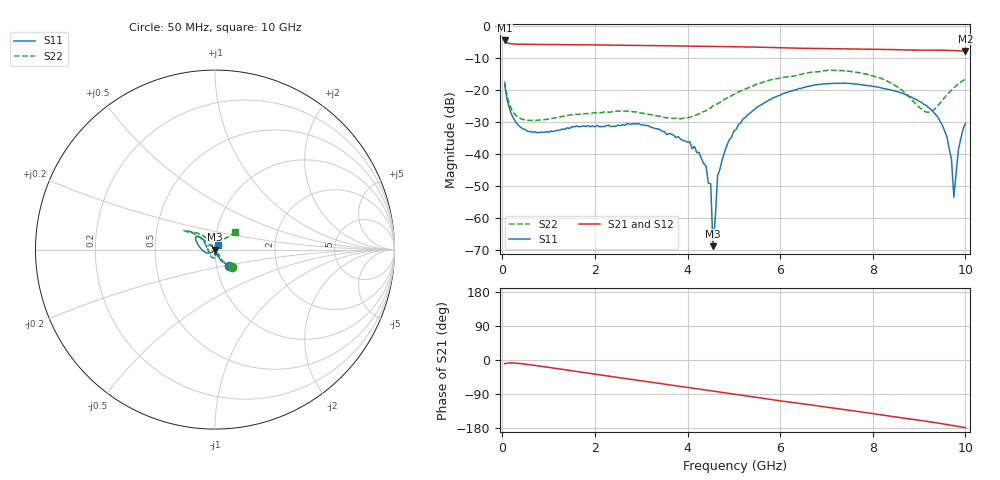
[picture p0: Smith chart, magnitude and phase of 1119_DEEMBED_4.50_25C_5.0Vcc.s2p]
!Hittite Microwave Corp.
!Digital Attenuator/PhaseShifter Rev 1.4.0
!Filename: C:\DATA\DATA\1119_DEEMBED_4.50_25C_5.0Vcc.s2p
!VNA ID: Agilent Technologies,N5224A,MY51441122,A.10.45.03
!Device type:
!2 Port Calibration.
!Temp(C): 25
!Lot Number:
!Serial Number:
!Operator:
!Misc:
!Attenuator:  4.500
# GHZ S DB R 50.0
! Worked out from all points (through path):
!   200 points, 50 MHz to 10 GHz, reference 50 ohm
!   highest |S21| = -4.50 dB at 50 MHz (marker M1); lowest = -7.8 dB at 10 GHz (marker M2)
!   group delay of S21, straight-line fit = 48.3 ps
!   lowest |S11| = -68.9 dB at 4.55 GHz (marker M3), VSWR 1.00, Z = 50 - j0.033 ohm
!   |S11| at or under -10 dB: start of sweep to end of sweep
!   |S22| runs from -29.5 to -13.8 dB; largest |S21 - S12| = 0.0013
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0.05  -18.28 -48.8  -4.50 -9.7  -4.50 -9.7  -17.41 -45.3
0.2  -27.69 -63.4  -5.56 -7.7  -5.56 -7.7  -26.08 -55.2
0.55  -33.00 -58.9  -5.71 -11.8  -5.71 -11.8  -29.51 -50.6
1.75  -31.23 -86.9  -5.86 -32.7  -5.86 -32.8  -27.43 -79.5
3.4  -32.36 -83.0  -6.13 -61.8  -6.14 -61.9  -28.22 -135.8
4.05  -36.24 -68.5  -6.27 -73.3  -6.28 -73.4  -28.56 -174.3
4.4  -43.79 -64.5  -6.35 -79.5  -6.37 -79.6  -26.47 162.2
4.45  -49.20 -49.4  -6.37 -80.4  -6.39 -80.5  -25.94 159.6
4.5  -49.36 -61.2  -6.38 -81.2  -6.40 -81.3  -25.64 156.9
4.55  -68.88 -113.4  -6.39 -82.1  -6.41 -82.1  -24.94 154.6
4.65  -46.85 123.5  -6.40 -83.8  -6.42 -83.9  -24.29 150.2
5.05  -32.38 131.7  -6.47 -90.8  -6.49 -90.9  -21.02 141.6
5.75  -23.20 139.0  -6.68 -103.3  -6.69 -103.4  -17.02 142.8
6.7  -18.60 142.1  -6.98 -119.2  -6.99 -119.2  -14.40 147.4
8.35  -19.86 161.6  -7.34 -147.7  -7.35 -147.7  -17.47 136.4
9.15  -24.76 -165.0  -7.51 -161.5  -7.53 -161.5  -26.88 104.4
9.400001  -28.37 -151.2  -7.54 -166.2  -7.55 -166.3  -25.03 65.1
9.6  -34.56 -137.4  -7.60 -170.3  -7.62 -170.3  -21.52 48.0
9.7  -41.65 -119.5  -7.65 -172.3  -7.66 -172.3  -20.04 44.1
9.75  -53.57 -38.6  -7.67 -173.3  -7.68 -173.3  -19.33 43.2
9.85  -38.66 44.0  -7.73 -175.4  -7.73 -175.4  -18.06 42.2
10  -30.47 51.1  -7.82 -178.4  -7.82 -178.4  -16.62 41.3
